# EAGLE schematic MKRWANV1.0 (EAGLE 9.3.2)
Assembly variants: Chip Antenna, Antenna Connector

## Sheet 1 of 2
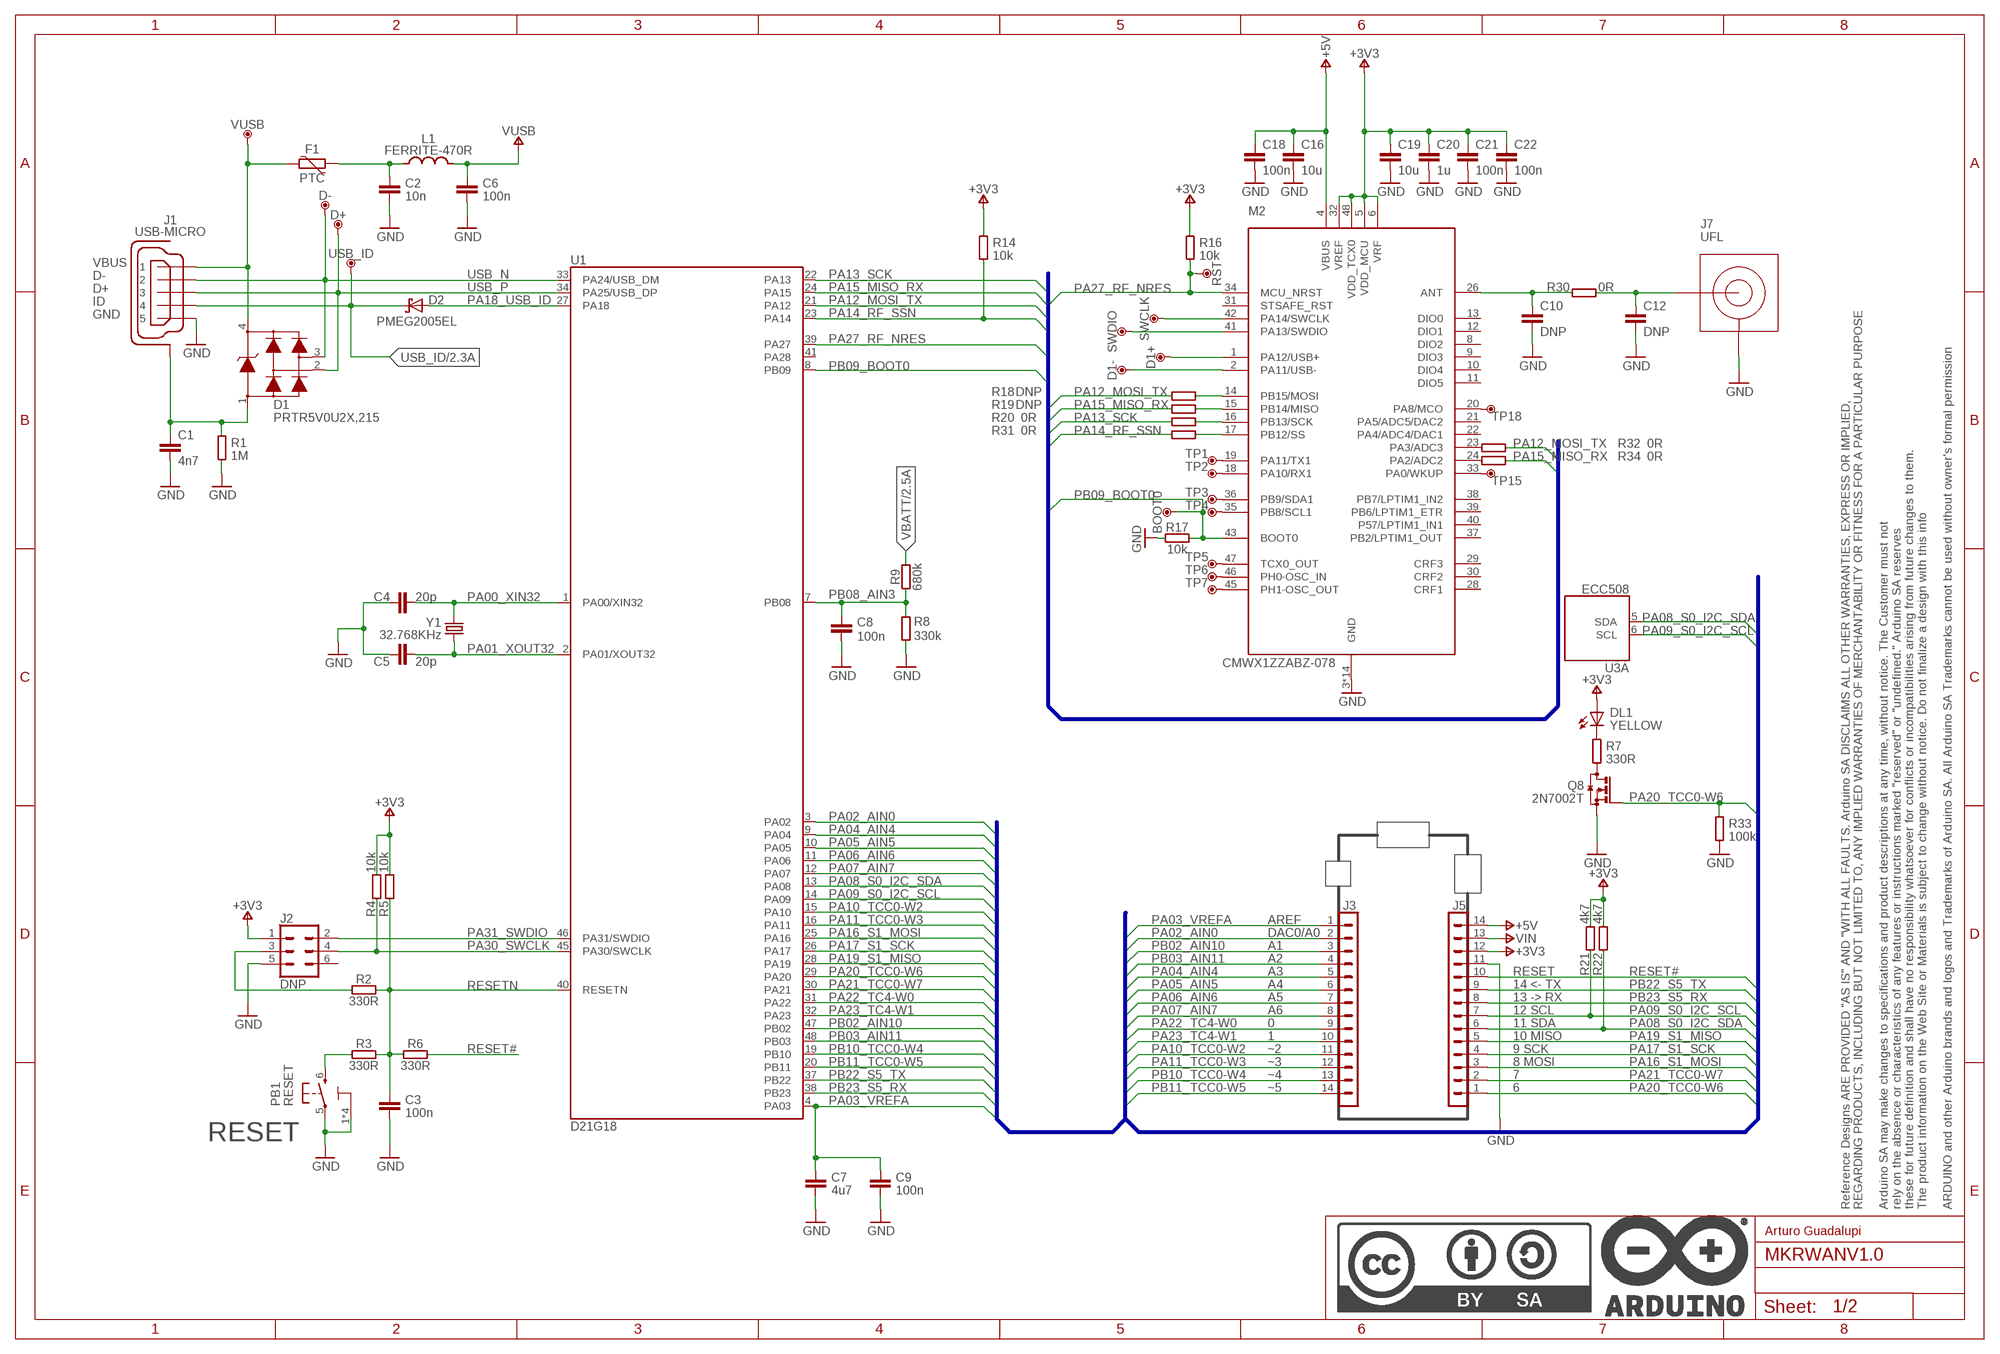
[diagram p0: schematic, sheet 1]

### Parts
BOOT0  DNP  TPTP-1.00MM  [TP-1.00MM]
C1  4n7  C4.7NF-0805  [0805-R2013X50N]
C2  10n  C-10NF-0402  [0402-1005X55N]
C3  100n  C-100NF-0402  [0402-1005X55N]
C4  20p  C-20PF-0402  [0402-1005X55N]
C5  20p  C-20PF-0402  [0402-1005X55N]
C6  100n  C-100NF-0402  [0402-1005X55N]
C7  4u7  C-4.7UF-0402  [0402-1005X55N]
C8  100n  C-100NF-0402  [0402-1005X55N]
C9  100n  C-100NF-0402  [0402-1005X55N]
C10  DNP  CDNP-0402  [0402-1005X55N]
C12  DNP  CDNP-0402  [0402-1005X55N]
C16  10u  C-10UF-0603  [0603-1608X90N]
C18  100n  C-100NF-0402  [0402-1005X55N]
C19  10u  C-10UF-0603  [0603-1608X90N]
C20  1u  C-1UF-0402  [0402-1005X55N]
C21  100n  C-100NF-0402  [0402-1005X55N]
C22  100n  C-100NF-0402  [0402-1005X55N]
D1  PRTR5V0U2X,215  [SOT190P230X110-4N]
D1+  DNP  TPTP-1.00MM  [TP-1.00MM]
D1-  DNP  TPTP-1.00MM  [TP-1.00MM]
D2  PMEG2005EL  [SODFL1008X40N-882D]
D+  DNP  TPTP-1.00MM  [TP-1.00MM]
D-  DNP  TPTP-1.00MM  [TP-1.00MM]
DL1  YELLOW  LED-YELLOW-0603  [LEDC1608X80N-AK]
F1  PTC  [0603-1608X90N]
FRAME1  DNP  A3-FRAME  [FRAME]
J1  USB-MICRO  [ZX62-AB-5PA]
J2  DNP  2X3_SMD_MALE  [2X3_SMT]
J3  DNP  PINHD-1X14-SMTH-SMD  [1X14_SMD_TH]
J5  DNP  PINHD-1X14-SMTH-SMD  [1X14_SMD_TH]
J7  UFL  [U.FL-R-SMT-1(60)]
L1  FERRITE-470R  [0603-1608X90N@1]
M2  CMWX1ZZABZ-078  [CMWX1ZZABZ-078]
PB1  RESET  TACTILE1  [C&K_PTS820_NO_HOLES]
Q8  2N7002T  [SOTFL50P160X78-3]
R1  1M  R-1M-0402  [0402-1005X55N]
R2  330R  R-330R-0402  [0402-1005X55N]
R3  330R  R-330R-0402  [0402-1005X55N]
R4  10k  R-10K-0402  [0402-1005X55N]
R5  10k  R-10K-0402  [0402-1005X55N]
R6  330R  R-330R-0402  [0402-1005X55N]
R7  330R  R-330R-0402  [0402-1005X55N]
R8  330k  R-330K-0402  [0402-1005X55N]
R9  680k  R-680K-0402  [0402-1005X55N]
R14  10k  R-10K-0402  [0402-1005X55N]
R16  10k  R-10K-0402  [0402-1005X55N]
R17  10k  R-10K-0402  [0402-1005X55N]
R18  DNP  R-DNP-0402  [0402-1005X55N]
R19  DNP  R-DNP-0402  [0402-1005X55N]
R20  0R  R-0R-0402  [0402-1005X55N]
R21  4k7  R-4K7-0402  [0402-1005X55N]
R22  4k7  R-4K7-0402  [0402-1005X55N]
R30  0R  R-0R-0402  [0402-1005X55N]
R31  0R  R-0R-0402  [0402-1005X55N]
R32  0R  R-0R-0402  [0402-1005X55N]
R33  100k  R-100K-0402  [0402-1005X55N]
R34  0R  R-0R-0402  [0402-1005X55N]
RST  DNP  TPTP-1.00MM  [TP-1.00MM]
SWCLK  DNP  TPTP-1.00MM  [TP-1.00MM]
SWDIO  DNP  TPTP-1.00MM  [TP-1.00MM]
TP1  DNP  TPTP-0.5MM  [TP-0.50MM]
TP2  DNP  TPTP-0.5MM  [TP-0.50MM]
TP3  DNP  TPTP-0.5MM  [TP-0.50MM]
TP4  DNP  TPTP-0.5MM  [TP-0.50MM]
TP5  DNP  TPTP-0.5MM  [TP-0.50MM]
TP6  DNP  TPTP-0.5MM  [TP-0.50MM]
TP7  DNP  TPTP-0.5MM  [TP-0.50MM]
TP15  DNP  TPTP-0.5MM  [TP-0.50MM]
TP18  DNP  TPTP-0.5MM  [TP-0.50MM]
U1  D21G18  ATSAMD21G18A-48QFN  [QFN50P700X700X90-49XN-EPSQ515]
U3  ECC508  ATECC508A-MAHDA-T8-UDFN  [SON50P300X200X60-9N-EP160X140]
USB_ID  DNP  TPTP-1.00MM  [TP-1.00MM]
VUSB  DNP  TPTP-1.00MM  [TP-1.00MM]
Y1  32.768KHz  32.768KHZ  [ABS07]

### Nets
+3V3: C19.1 C20.1 C21.1 C22.1 DL1.A J2.1 J5.12 M2.5(VDD_MCU) M2.6(VRF) M2.32(VREF) M2.48(VDD_TCX0) R4.2 R5.2 R14.2 R16.2 R21.2 R22.2 ; also sheet 2
+5V: C16.1 C18.1 J5.14 M2.4(VBUS) ; also sheet 2
GND: C1.2 C2.2 C3.2 C4.1 C5.1 C6.2 C7.2 C8.2 C9.2 C10.2 C12.2 C16.2 C18.2 C19.2 C20.2 C21.2 C22.2 J1.5 J2.5 J5.11 J7.GND1(GND) J7.GND2(GND) M2.3(GND) M2.7(GND) M2.25(GND) M2.27(GND) M2.44(GND) M2.49(GND) M2.50(GND) M2.51(GND) M2.52(GND) M2.53(GND) M2.54(GND) M2.55(GND) M2.56(GND) M2.57(GND) PB1.1 PB1.2 PB1.3 PB1.4 PB1.5 Q8.S R1.1 R8.1 R17.1 R33.1 ; also sheet 2
N17650912: D1.4 F1.2 J1.1 VUSB.X
N17658775: PB1.6 R3.1
N$1: C1.1 D1.1 J1.6(SH) J1.7(SH) J1.8(SH) J1.9(SH) J1.10(SH) J1.11(SH) R1.2
N$2: C2.1 F1.1 L1.1
N$3: DL1.C R7.2
N$4: J2.3 R2.1
N$5: M2.24(PA2/ADC2) R34.1
N$6: Q8.D R7.1
N$7: M2.23(PA3/ADC3) R32.1
N$9: M2.19(PA11/TX1) TP1.X
N$10: M2.14(PB15/MOSI) R18.1
N$11: M2.15(PB14/MISO) R19.1
N$13: M2.16(PB13/SCK) R20.1
N$14: M2.17(PB12/SS) R31.1
N$15: M2.41(PA13/SWDIO) SWDIO.X
N$16: M2.42(PA14/SWCLK) SWCLK.X
N$17: C12.1 J7.SIG R30.2
N$18: D1+.X M2.1(PA12/USB+)
N$19: D1-.X M2.2(PA11/USB-)
N$20: M2.18(PA10/RX1) TP2.X
N$21: M2.36(PB9/SDA1) TP3.X
N$22: M2.35(PB8/SCL1) TP4.X
N$23: M2.47(TCX0_OUT) TP5.X
N$24: M2.46(PH0-OSC_IN) TP6.X
N$25: M2.45(PH1-OSC_OUT) TP7.X
N$33: M2.33(PA0/WKUP) TP15.X
N$36: M2.20(PA8/MCO) TP18.X
N$38: C10.1 M2.26(ANT) R30.1
PA00_XIN32: C4.2 U1.1(PA00/XIN32) Y1.2
PA01_XOUT32: C5.2 U1.2(PA01/XOUT32) Y1.1
PA02_AIN0: J3.2 U1.3(PA02)
PA03_VREFA: C7.1 C9.1 J3.1 U1.4(PA03)
PA04_AIN4: J3.5 U1.9(PA04)
PA05_AIN5: J3.6 U1.10(PA05)
PA06_AIN6: J3.7 U1.11(PA06)
PA07_AIN7: J3.8 U1.12(PA07)
PA08_S0_I2C_SDA: J5.6 R22.1 U1.13(PA08) U3.5(A:SDA)
PA09_S0_I2C_SCL: J5.7 R21.1 U1.14(PA09) U3.6(A:SCL)
PA10_TCC0-W2: J3.11 U1.15(PA10)
PA11_TCC0-W3: J3.12 U1.16(PA11)
PA12_MOSI_TX: R18.2 R32.2 U1.21(PA12)
PA13_SCK: R20.2 U1.22(PA13)
PA14_RF_SSN: R14.1 R31.2 U1.23(PA14)
PA15_MISO_RX: R19.2 R34.2 U1.24(PA15)
PA16_S1_MOSI: J5.3 U1.25(PA16)
PA17_S1_SCK: J5.4 U1.26(PA17)
PA18_USB_ID: D2.A U1.27(PA18)
PA19_S1_MISO: J5.5 U1.28(PA19)
PA20_TCC0-W6: J5.1 Q8.G R33.2 U1.29(PA20)
PA21_TCC0-W7: J5.2 U1.30(PA21)
PA22_TC4-W0: J3.9 U1.31(PA22)
PA23_TC4-W1: J3.10 U1.32(PA23)
PA27_RF_NRES: M2.34(MCU_NRST) R16.1 RST.X U1.39(PA27)
PA30_SWCLK: J2.4 R4.1 U1.45(PA30/SWCLK)
PA31_SWDIO: J2.2 U1.46(PA31/SWDIO)
PB02_AIN10: J3.3 U1.47(PB02)
PB03_AIN11: J3.4 U1.48(PB03)
PB08_AIN3: C8.1 R8.2 R9.1 U1.7(PB08)
PB09_BOOT0: BOOT0.X M2.43(BOOT0) R17.2 U1.8(PB09)
PB10_TCC0-W4: J3.13 U1.19(PB10)
PB11_TCC0-W5: J3.14 U1.20(PB11)
PB22_S5_TX: J5.9 U1.37(PB22)
PB23_S5_RX: J5.8 U1.38(PB23)
RESET#: J5.10 R6.2
RESETN: C3.1 R2.2 R3.2 R5.1 R6.1 U1.40(RESETN)
USB_ID: D2.C J1.4 USB_ID.X ; also sheet 2
USB_N: D1.3 D-.X J1.2 U1.33(PA24/USB_DM)
USB_P: D1.2 D+.X J1.3 U1.34(PA25/USB_DP)
VBATT: R9.2 ; also sheet 2
VIN: J5.13 ; also sheet 2
VUSB: C6.1 L1.2 ; also sheet 2
Unconnected: J2.6 M2.8(DIO2) M2.9(DIO3) M2.10(DIO4) M2.11(DIO5) M2.12(DIO1) M2.13(DIO0) M2.21(PA5/ADC5/DAC2) M2.22(PA4/ADC4/DAC1) M2.28(CRF1) M2.29(CRF3) M2.30(CRF2) M2.31(STSAFE_RST) M2.37(PB2/LPTIM1_OUT) M2.38(PB7/LPTIM1_IN2) M2.39(PB6/LPTIM1_ETR) M2.40(P57/LPTIM1_IN1) U1.41(PA28)

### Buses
PA03_VREFA,PA02_AIN0,PB02_AIN10,PB03_AIN11,PA04_AIN4,PA05_AIN5,PA06_AIN6,PA07_AIN7,PA22_TC4-W0,PA23_TC4-W1,PA10_TCC0-W2,PA11_TCC0-W3,PB10_TCC0-W4,PB11_TCC0-W5,PA20_TCC0-W6,PA21_TCC0-W7,PA16_S1_MOSI,PA17_S1_SCK,PA19_S1_MISO,PA08_S0_I2C_SDA,PA09_S0_I2C_SCL,PB23_S5_RX,PB22_S5_TX,RESET#
B$1

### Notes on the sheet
- AREF
- DAC0/A0
- A1
- A2
- A3 | RESET
- A4 | 14 <- TX
- A5 | 13 -> RX
- A6 | 12 SCL
- 0 | 11 SDA
- 1 | 10 MISO
- ~2 | 9 SCK
- ~3 | 8 MOSI
- ~4 | 7
- ~5 | 6
- RESET
- Arturo Guadalupi

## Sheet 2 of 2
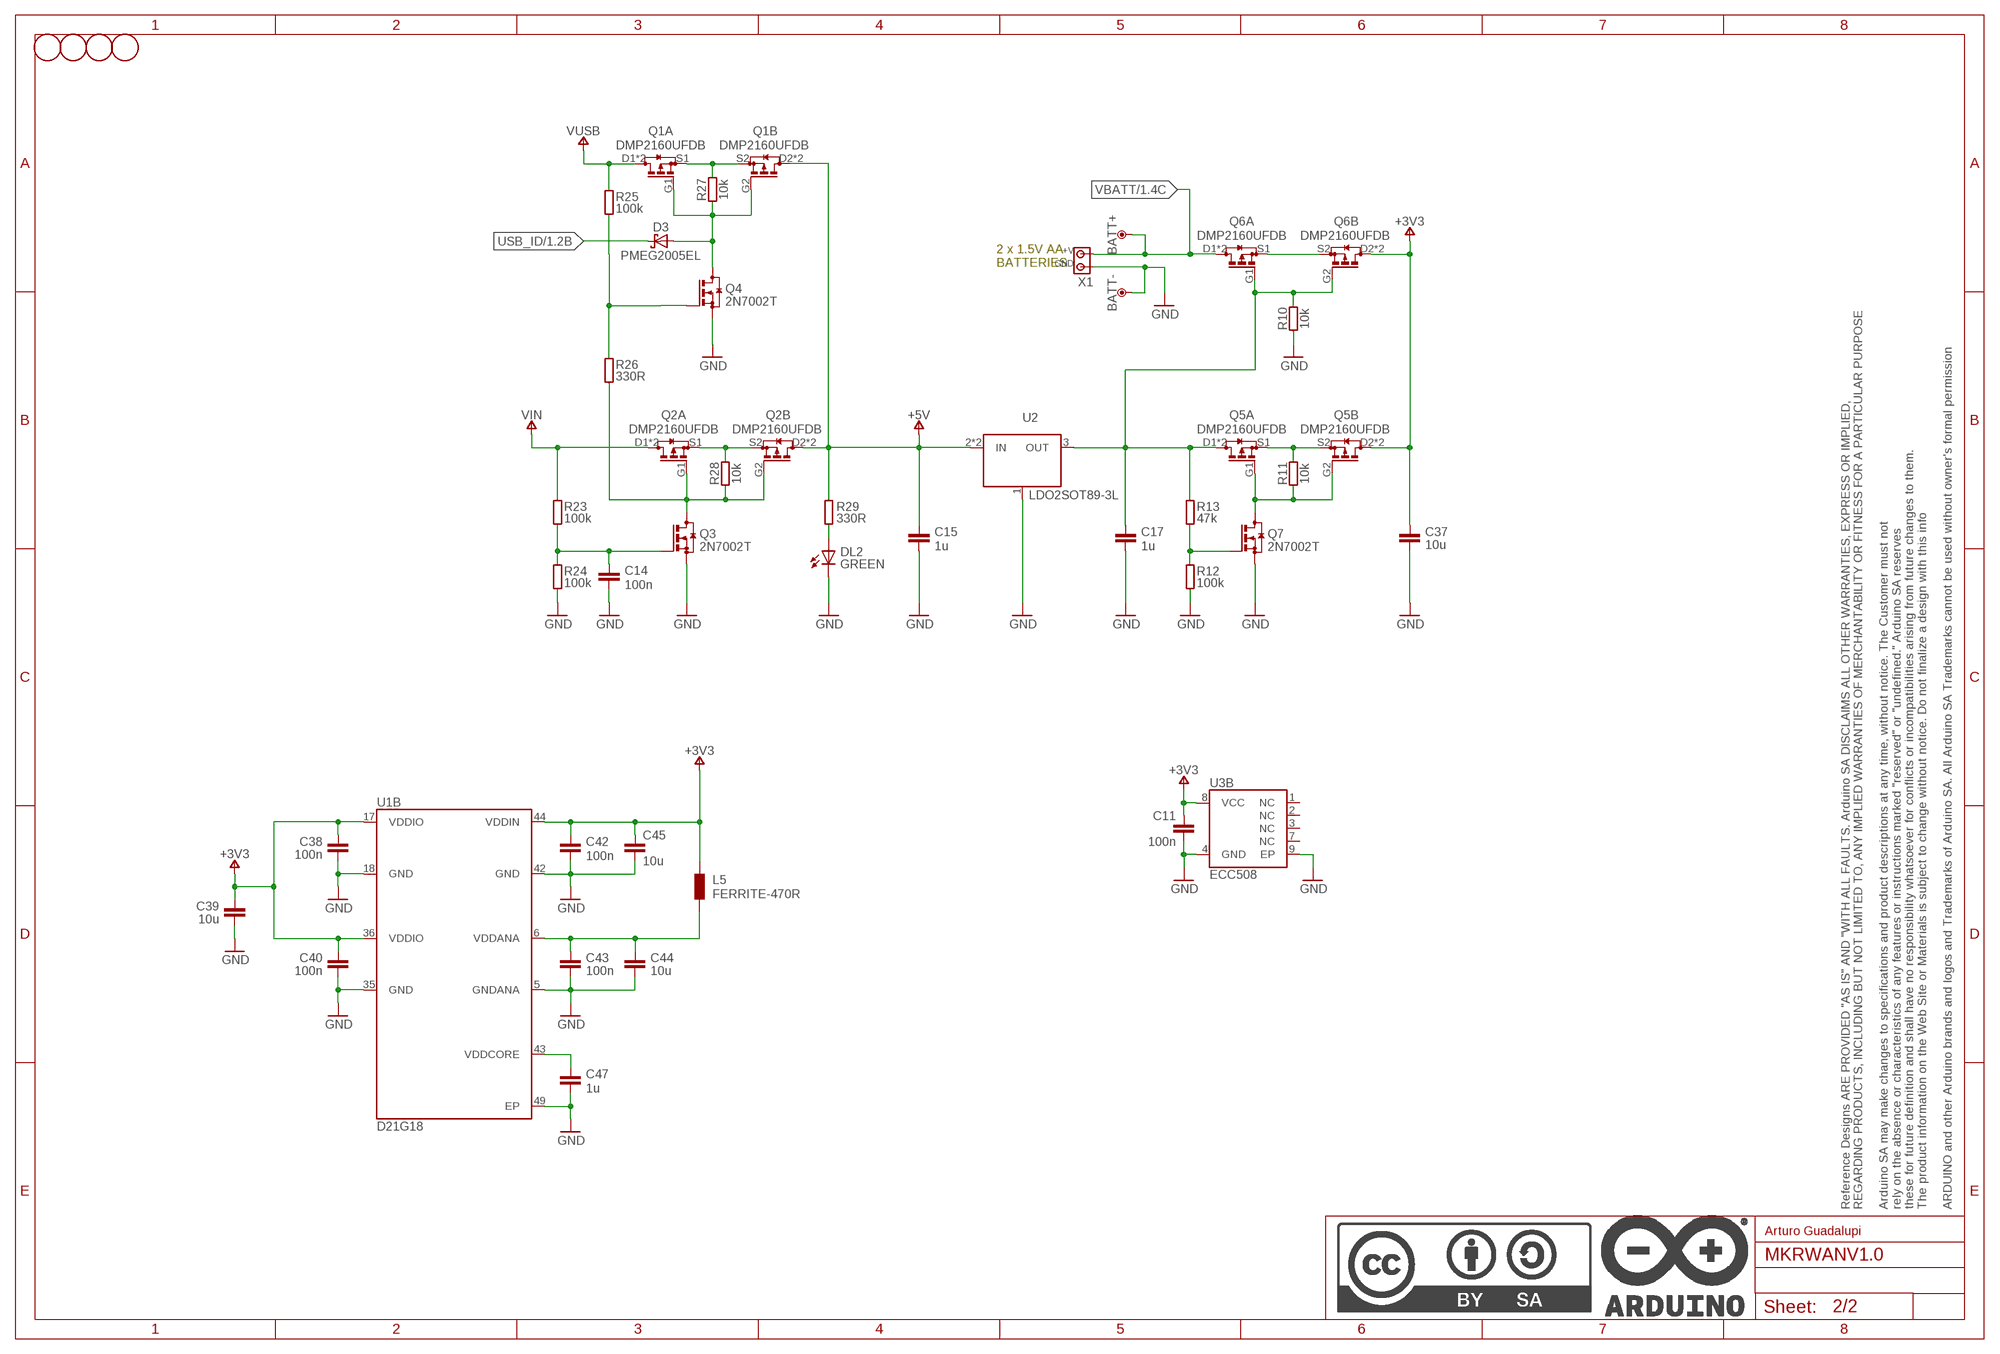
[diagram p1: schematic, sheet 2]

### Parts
BATT+  DNP  TPTP-1.00MM  [TP-1.00MM]
BATT-  DNP  TPTP-1.00MM  [TP-1.00MM]
C11  100n  C-100NF-0402  [0402-1005X55N]
C14  100n  C-100NF-0402  [0402-1005X55N]
C15  1u  C-1UF-0402  [0402-1005X55N]
C17  1u  C-1UF-0402  [0402-1005X55N]
C37  10u  C-10UF-0603  [0603-1608X90N]
C38  100n  C-100NF-0402  [0402-1005X55N]
C39  10u  C-10UF-0603  [0603-1608X90N]
C40  100n  C-100NF-0402  [0402-1005X55N]
C42  100n  C-100NF-0402  [0402-1005X55N]
C43  100n  C-100NF-0402  [0402-1005X55N]
C44  10u  C-10UF-0603  [0603-1608X90N]
C45  10u  C-10UF-0603  [0603-1608X90N]
C47  1u  C-1UF-0402  [0402-1005X55N]
D3  PMEG2005EL  [SODFL1008X40N-882D]
DL2  GREEN  LED-GREEN-0603  [LEDC1608X80N-AK]
FD1  DNP  FIDUCIAL-1.5MM  [FD-1-1.5]
FD2  DNP  FIDUCIAL-1.5MM  [FD-1-1.5]
FD3  DNP  FIDUCIAL-1.5MM  [FD-1-1.5]
FD4  DNP  FIDUCIAL-1.5MM  [FD-1-1.5]
FRAME2  DNP  A3-FRAME  [FRAME]
L5  FERRITE-470R  [0603-1608X90N@1]
Q1  DMP2160UFDB  [PWR_SC70]
Q2  DMP2160UFDB  [PWR_SC70]
Q3  2N7002T  [SOTFL50P160X78-3]
Q4  2N7002T  [SOTFL50P160X78-3]
Q5  DMP2160UFDB  [PWR_SC70]
Q6  DMP2160UFDB  [PWR_SC70]
Q7  2N7002T  [SOTFL50P160X78-3]
R10  10k  R-10K-0402  [0402-1005X55N]
R11  10k  R-10K-0402  [0402-1005X55N]
R12  100k  R-100K-0402  [0402-1005X55N]
R13  47k  R-47K-0402  [0402-1005X55N]
R23  100k  R-100K-0402  [0402-1005X55N]
R24  100k  R-100K-0402  [0402-1005X55N]
R25  100k  R-100K-0402  [0402-1005X55N]
R26  330R  R-330R-0402  [0402-1005X55N]
R27  10k  R-10K-0402  [0402-1005X55N]
R28  10k  R-10K-0402  [0402-1005X55N]
R29  330R  R-330R-0402  [0402-1005X55N]
U2  LDO2SOT89-3L  [SOT89-3L]
X1  SCREW2X2.54  [SCREW2]

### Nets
+3V3: C11.1 C37.1 C38.1 C39.1 C40.1 C42.1 C45.1 L5.1 Q5.D2'(B:D) Q5.D2(B:D) Q6.D2'(B:D) Q6.D2(B:D) U1.17(VDDIO) U1.36(VDDIO) U1.44(VDDIN) U3.8(B:VCC) ; also sheet 1
+5V: C15.1 Q1.D2'(B:D) Q1.D2(B:D) Q2.D2'(B:D) Q2.D2(B:D) R29.2 U2.2(IN) U2.TH(IN) ; also sheet 1
GND: BATT-.X C11.2 C14.2 C15.2 C17.2 C37.2 C38.2 C39.2 C40.2 C42.2 C43.2 C44.2 C45.2 C47.2 DL2.C Q3.S Q4.S Q7.S R10.1 R12.1 R24.1 U1.5(GNDANA) U1.18(GND) U1.35(GND) U1.42(GND) U1.49(EP) U2.1(GND/ADJ) U3.4(B:GND) U3.9(B:EP) X1.GND ; also sheet 1
N1: Q5.S1(A:S) Q5.S2(B:S) R11.2
N2: Q5.G1(A:G) Q5.G2(B:G) Q7.D R11.1
N3: Q7.G R12.2 R13.1
N17690335: Q1.S1(A:S) Q1.S2(B:S) R27.2
N17690346: D3.A Q1.G1(A:G) Q1.G2(B:G) Q4.D R27.1
N17690381: Q4.G R25.1 R26.2
N17690821: Q2.S1(A:S) Q2.S2(B:S) R28.2
N17690840: Q2.G1(A:G) Q2.G2(B:G) Q3.D R26.1 R28.1
N17690878: C14.1 Q3.G R23.1 R24.2
N17834267: DL2.A R29.1
N17852357: C43.1 C44.1 L5.2 U1.6(VDDANA)
N$8: C17.1 Q5.D1'(A:D) Q5.D1(A:D) Q6.G1(A:G) Q6.G2(B:G) R10.2 R13.2 U2.3(OUT)
N$12: Q6.S1(A:S) Q6.S2(B:S)
N$46: C47.1 U1.43(VDDCORE)
USB_ID: D3.C ; also sheet 1
VBATT: BATT+.X Q6.D1'(A:D) Q6.D1(A:D) X1.V+ ; also sheet 1
VIN: Q2.D1'(A:D) Q2.D1(A:D) R23.2 ; also sheet 1
VUSB: Q1.D1'(A:D) Q1.D1(A:D) R25.2 ; also sheet 1
Unconnected: U3.1(B:NC) U3.2(B:NC) U3.3(B:NC) U3.7(B:NC)

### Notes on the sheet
- 2 x 1.5V AA
  BATTERIES
- Arturo Guadalupi

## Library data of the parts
BATT+ BATT- BOOT0 D1+ D1- D+ D- RST SWCLK SWDIO TP1-TP7 TP15 TP18 USB_ID VUSB = Arduino-utility:TP: Testpoint; DATASHEET: DNP; DISTRIBUTOR-LINK: DNP; DISTRIBUTOR-PN: DNP; MANUFACTURER: DNP; MANUFACTURER-PN: DNP
C1 = Arduino-rcl:C: SMD Capacitor; DATASHEET: http://www.kemet.com/Lists/ProductCatalog/Attachments/40/KEM_C1010_X7R_HV_SMD.pdf; DISTRIBUTOR-LINK: www.kemet.com/docfinder?Partnumber=C0805C472KDRACTU; DISTRIBUTOR-PN: 399-6738-1-ND; MANUFACTURER: Kemet; MANUFACTURER-PN: C0805C472KDRACTU
C2 = Arduino-rcl:C: SMD Capacitor; DATASHEET: http://search.murata.co.jp/Ceramy/image/img/A01X/partnumbering_e_01.pdf; DISTRIBUTOR-LINK: http://www.digikey.com/product-detail/en/murata-electronics-north-america/GRM155R71H103KA88J/490-6351-1-ND/3845548; DISTRIBUTOR-PN: 490-6351-1-ND; MANUFACTURER: Murata; MANUFACTURER-PN: GRM155R71H103KA88J
C3 C6 C8 C9 C11 C14 C18 C21 C22 C38 C40 C42 C43 = Arduino-rcl:C: SMD Capacitor; DATASHEET: http://www.tdk.com/pdf/TDKMLCCCapRange.pdf; DISTRIBUTOR-LINK: http://www.digikey.com/product-detail/en/tdk-corporation/C1005X5R1H104K050BB/445-5942-1-ND/2443982; DISTRIBUTOR-PN: 445-5942-1-ND; MANUFACTURER: TDK; MANUFACTURER-PN: C1005X5R1H104K050BB
C4 C5 = Arduino-rcl:C: SMD Capacitor; DATASHEET: http://www.kemet.com/docfinder?Partnumber=CBR04C200J5GAC; DISTRIBUTOR-LINK: http://www.digikey.com/product-detail/en/kemet/CBR04C200J5GAC/399-6173-1-ND/2732143; DISTRIBUTOR-PN: 399-6173-1-ND; MANUFACTURER: Kemet; MANUFACTURER-PN: CBR04C200J5GAC
C7 = Arduino-rcl:C: SMD Capacitor; DATASHEET: http://search.murata.co.jp/Ceramy/image/img/A01X/partnumbering_e_01.pdf; DISTRIBUTOR-LINK: http://www.digikey.com/product-detail/en/murata-electronics-north-america/GRM155R60J475ME47D/490-5915-1-ND/3719860; DISTRIBUTOR-PN: 490-5915-1-ND; MANUFACTURER: Murata; MANUFACTURER-PN: GRM155R60J475ME47D
C10 C12 = Arduino-rcl:C: SMD Capacitor; DATASHEET: DNP; DISTRIBUTOR-LINK: DNP; DISTRIBUTOR-PN: DNP; MANUFACTURER: DNP; MANUFACTURER-PN: DNP
C15 C17 C20 C47 = Arduino-rcl:C: SMD Capacitor; DATASHEET: http://search.murata.co.jp/Ceramy/image/img/A01X/partnumbering_e_01.pdf; DISTRIBUTOR-LINK: http://www.digikey.com/product-detail/en/murata-electronics-north-america/GRM155R61E105KA12D/490-10017-1-ND/5026367; DISTRIBUTOR-PN: 490-10017-1-ND; MANUFACTURER: Murata; MANUFACTURER-PN: GRM155R61E105KA12D
C16 C19 C37 C39 C44 C45 = Arduino-rcl:C: SMD Capacitor; DATASHEET: http://www.murata.com/~/media/webrenewal/support/library/catalog/products/capacitor/mlcc/c02e.pdf; DISTRIBUTOR-LINK: http://www.digikey.com/product-search/en?keywords=490-10728-1-ND; DISTRIBUTOR-PN: 490-10728-1-ND; MANUFACTURER: Murata; MANUFACTURER-PN: GRM188R61C106KAALD
D1 = Arduino-diodes:PRTR5V0U2X,215: USB ESD protection; DATASHEET: http://www.nxp.com/documents/data_sheet/PRTR5V0U2X.pdf; DISTRIBUTOR-LINK: http://www.digikey.com/product-detail/en/nxp-semiconductors/PRTR5V0U2X,215/568-4140-1-ND/1589981; DISTRIBUTOR-PN: 568-4140-1-ND; MANUFACTURER: NXP; MANUFACTURER-PN: PRTR5V0U2X,215
D2 D3 = Arduino-diodes:PMEG2005EL: DIODE SCHOTTKY 20V 500MA SOD882; DATASHEET: http://www.nxp.com/documents/data_sheet/PMEG2005EL.pdf; DISTRIBUTOR-LINK: http://www.digikey.com/product-detail/en/nxp-semiconductors/PMEG2005EL,315/568-6754-1-ND/2676794; DISTRIBUTOR-PN: 568-6754-1-ND; MANUFACTURER: NXP; MANUFACTURER-PN: PMEG2005EL,315
DL1 = Arduino-diodes:LED: LED; DATASHEET: http://media.digikey.com/pdf/Data%20Sheets/Avago%20PDFs/HSMz-Czzz.pdf; DISTRIBUTOR-LINK: http://www.digikey.com/product-detail/en/broadcom-limited/HSMY-C190/516-1424-1-ND/637748; DISTRIBUTOR-PN: 516-1424-1-ND; MANUFACTURER: Avago; MANUFACTURER-PN: HSMY-C190
DL2 = Arduino-diodes:LED: LED; DATASHEET: http://media.digikey.com/pdf/Data%20Sheets/Avago%20PDFs/HSMz-Czzz.pdf; DISTRIBUTOR-LINK: http://www.digikey.com/product-detail/en/broadcom-limited/HSMG-C190/516-1425-1-ND/637749; DISTRIBUTOR-PN: 516-1425-1-ND; MANUFACTURER: Avago; MANUFACTURER-PN: HSMG-C190
F1 = Arduino-rcl:PTC: SMD PTC; DATASHEET: http://www.bourns.com/docs/Product-Datasheets/mffsmf.pdf; DISTRIBUTOR-LINK: http://www.digikey.com/product-detail/en/bourns-inc/MF-FSMF050X-2/MF-FSMF050X-2CT-ND/2039389; DISTRIBUTOR-PN: MF-FSMF050X-2CT-ND; MANUFACTURER: Bourns Inc; MANUFACTURER-PN: MF-FSMF050X-2
FD1-FD4 = Arduino-utility:FIDUCIAL: Fiducial mount; DATASHEET: DNP; DISTRIBUTOR-LINK: DNP; DISTRIBUTOR-PN: DNP; MANUFACTURER: DNP; MANUFACTURER-PN: DNP
FRAME1 FRAME2 = Arduino-utility:A3-FRAME; CODE-ARDUINO: DNP; DATASHEET: DNP; DISTRIBUTOR-LINK: DNP; DISTRIBUTOR-PN: DNP; MANUFACTURER: DNP; MANUFACTURER-PN: DNP; NOTE: DNP
J1 = Arduino-connectors:USB-MICRO: USB - micro AB USB 2.0 Receptacle Connector 5 Position Surface Mount, Right Angle, Horizontal; DATASHEET: https://www.hirose.com/product/en/download_file/key_name/ZX/category/Catalog/doc_file_id/31704/?file_category_id=4&item_id=13&is_series=1; DISTRIBUTOR-LINK: http://www.digikey.com/product-detail/en/hirose-electric-co-ltd/ZX62-AB-5PA(31)/H125279CT-ND/5994741; DISTRIBUTOR-PN: H125279CT-ND; MANUFACTURER: Hirose; MANUFACTURER-PN: ZX62-AB-5PA(31)
J2 = Arduino-connectors:2X3_SMD_MALE: SMD connector; DATASHEET: DNP; DISTRIBUTOR-LINK: DNP; DISTRIBUTOR-PN: DNP; MANUFACTURER: DNP; MANUFACTURER-PN: DNP
J3 J5 = Arduino-connectors:PINHD-1X14-SM: PIN HEADER; DATASHEET: -; DISTRIBUTOR-LINK: -; DISTRIBUTOR-PN: -; MANUFACTURER: ELDECO; MANUFACTURER-PN: FH254114DF08500T
J7 = Arduino-connectors:UFL: U.FL, Ultra Miniature Coaxial Connector Receptacle, Male Pin 50 Ohm Surface Mount Solder; DATASHEET: http://media.digikey.com/pdf/Data%20Sheets/Hirose%20PDFs/UFL%20Series.pdf; DISTRIBUTOR-LINK: http://www.digikey.com/product-search/en?keywords=U.FL-R-SMT-1(60); DISTRIBUTOR-PN: U.FL-R-SMT-1(60)-ND; MANUFACTURER: Hirose; MANUFACTURER-PN: U.FL-R-SMT-1(60)
L1 = Arduino-rcl:FERRITE-470R: FERRITE BEAD 470 OHM 0603 1LN; DATASHEET: http://search.murata.co.jp/Ceramy/image/img/PDF/ENG/L0110S0100BLM18P.pdf; DISTRIBUTOR-LINK: http://www.digikey.com/product-detail/en/murata-electronics-north-america/BLM18PG471SN1D/490-5223-1-ND/1948399; DISTRIBUTOR-PN: 490-5223-1-ND; MANUFACTURER: Murata; MANUFACTURER-PN: BLM18PG471SN1D
L5 = Arduino-rcl:FERRITE: FERRITE BEAD 470 OHM 0603 1LN; DATASHEET: http://search.murata.co.jp/Ceramy/image/img/PDF/ENG/L0110S0100BLM18P.pdf; DISTRIBUTOR-LINK: http://www.digikey.com/product-detail/en/murata-electronics-north-america/BLM18PG471SN1D/490-5223-1-ND/1948399; DISTRIBUTOR-PN: 490-5223-1-ND; MANUFACTURER: Murata; MANUFACTURER-PN: BLM18PG471SN1D
M2 = Arduino-ucs&SoCs:CMWX1ZZABZ-078; DATASHEET: https://www.arrow.altech.co.za/sites/arrow/files/Murata%20LoRa%20Module%20Preliminary%20Datasheet%20SP-ABZ-G.PDF; DISTRIBUTOR-LINK: https://www.digikey.com/product-detail/en/murata-electronics-north-america/CMWX1ZZABZ-078/490-16143-1-ND/6834151; DISTRIBUTOR-PN: 490-16143-1-ND; MANUFACTURER: Murata; MANUFACTURER-PN: CMWX1ZZABZ-078
PB1 = Arduino-pushbuttons:TACTILE1: Tactile Switch SPST-NO Top Actuated Surface Mount; DATASHEET: http://www.ckswitches.com/media/1474/pts820.pdf; DISTRIBUTOR-LINK: http://www.digikey.com/product-detail/en/c-k-components/PTS820%20J25K%20SMTR%20LFS/PTS820%20J25K%20SMTR%20LFS-ND/4142165; DISTRIBUTOR-PN: PTS820 J25K SMTR LFS-ND; MANUFACTURER: C&K; MANUFACTURER-PN: PTS820 J25K SMTR LFS
Q1 Q2 Q5 Q6 = Arduino-transistors:DMP2160UFDB: MOSFET 2P-CH 20V 3.8A 6UDFN; DATASHEET: http://www.diodes.com/_files/datasheets/ds31643.pdf; DISTRIBUTOR-LINK: http://www.digikey.com/product-detail/en/diodes-incorporated/DMP2160UFDB-7/DMP2160UFDB-7DI-ND/4249940; DISTRIBUTOR-PN: DMP2160UFDB-7DI-ND; MANUFACTURER: Diodes Inc; MANUFACTURER-PN: DMP2160UFDB-7
Q3 Q4 Q7 Q8 = Arduino-transistors:2N7002T: MOSFET N-CH 60V 115MA SOT-523; DATASHEET: http://www.diodes.com/_files/datasheets/ds30301.pdf; DISTRIBUTOR-LINK: http://www.digikey.com/product-detail/en/diodes-incorporated/2N7002T-7-F/2N7002T-FDICT-ND/815290; DISTRIBUTOR-PN: 2N7002T-FDICT-ND; MANUFACTURER: Diodes Incorporated; MANUFACTURER-PN: 2N7002T-7-F
R1 = Arduino-rcl:R: SMD Resistor; DATASHEET: www.yageo.com.tw/exep/pages/download/literatures/PYu-R_INT-thick_7.pdf; DISTRIBUTOR-LINK: http://www.digikey.com/product-detail/en/yageo/RC0402JR-07330RL/311-330JRCT-ND/729412; DISTRIBUTOR-PN: 311-330JRCT-ND; MANUFACTURER: Yageo; MANUFACTURER-PN: RC0402JR-07330RL
R2 R3 R6 R7 R26 R29 = Arduino-rcl:R: SMD Resistor; DATASHEET: www.yageo.com.tw/exep/pages/download/literatures/PYu-R_INT-thick_7.pdf; DISTRIBUTOR-LINK: http://www.digikey.com/product-detail/en/yageo/RC0402FR-07330RL/311-330LRCT-ND/729541; DISTRIBUTOR-PN: 311-330LRCT-ND; MANUFACTURER: Yageo; MANUFACTURER-PN: RC0402FR-07330RL
R4 R5 R10 R11 R14 R16 R17 R27 R28 = Arduino-rcl:R: SMD Resistor; DATASHEET: www.yageo.com.tw/exep/pages/download/literatures/PYu-R_INT-thick_7.pdf; DISTRIBUTOR-LINK: http://www.digikey.com/product-detail/en/yageo/RC0402FR-0710KL/311-10.0KLRCT-ND/729470; DISTRIBUTOR-PN: 311-10.0KLRCT-ND; MANUFACTURER: Yageo; MANUFACTURER-PN: RC0402FR-0710KL
R8 = Arduino-rcl:R: SMD Resistor; DATASHEET: www.yageo.com.tw/exep/pages/download/literatures/PYu-R_INT-thick_7.pdf; DISTRIBUTOR-LINK: http://www.digikey.com/product-detail/en/yageo/RC0402JR-07330KL/311-330KJRCT-ND/729413; DISTRIBUTOR-PN: 311-330KJRCT-ND; MANUFACTURER: Yageo; MANUFACTURER-PN: RC0402JR-07330KL
R9 = Arduino-rcl:R: SMD Resistor; DATASHEET: www.yageo.com.tw/exep/pages/download/literatures/PYu-R_INT-thick_7.pdf; DISTRIBUTOR-LINK: http://www.digikey.it/product-detail/it/yageo/RC0402JR-07680KL/311-680KJRTR-ND/726501; DISTRIBUTOR-PN: 311-680KJRTR-ND; MANUFACTURER: Yageo; MANUFACTURER-PN: RC0402JR-07680KL
R12 R23-R25 R33 = Arduino-rcl:R: SMD Resistor; DATASHEET: www.yageo.com.tw/exep/pages/download/literatures/PYu-R_INT-thick_7.pdf; DISTRIBUTOR-LINK: http://www.digikey.com/product-detail/en/yageo/RC0402FR-07100KL/311-100KLRCT-ND/729473; DISTRIBUTOR-PN: 311-100KLRCT-ND; MANUFACTURER: Yageo; MANUFACTURER-PN: RC0402FR-07100KL
R13 = Arduino-rcl:R: SMD Resistor; DATASHEET: www.yageo.com.tw/exep/pages/download/literatures/PYu-R_INT-thick_7.pdf; DISTRIBUTOR-LINK: http://www.digikey.com/product-detail/en/yageo/RC0402JR-0747KL/311-47KJRCT-ND/729432; DISTRIBUTOR-PN: 311-47KJRCT-ND; MANUFACTURER: Yageo; MANUFACTURER-PN: RC0402JR-0747KL
R18 R19 = Arduino-rcl:R: SMD Resistor; DATASHEET: DNP; DISTRIBUTOR-LINK: DNP; DISTRIBUTOR-PN: DNP; MANUFACTURER: DNP; MANUFACTURER-PN: DNP
R20 R30-R32 R34 = Arduino-rcl:R: SMD Resistor; DATASHEET: www.yageo.com.tw/exep/pages/download/literatures/PYu-R_INT-thick_7.pdf; DISTRIBUTOR-LINK: http://www.digikey.com/product-detail/en/yageo/RC0402FR-070RL/311-0.0LRCT-ND/2827888; DISTRIBUTOR-PN: 311-0.0LRCT-ND; MANUFACTURER: Yageo; MANUFACTURER-PN: RC0402FR-070RL
R21 R22 = Arduino-rcl:R: SMD Resistor; DATASHEET: www.yageo.com.tw/exep/pages/download/literatures/PYu-R_INT-thick_7.pdf; DISTRIBUTOR-LINK: http://www.digikey.com/product-detail/en/yageo/RC0402FR-074K7L/311-4.7KLRCT-ND/2827881; DISTRIBUTOR-PN: 311-4.7KLRCT-ND; MANUFACTURER: Yageo; MANUFACTURER-PN: RC0402FR-074K7L
U1 = Arduino-ucs&SoCs:ATSAMD21G18A-48: ARM® Cortex®-M0+ SAM D21G Microcontroller IC 32-Bit 48MHz 256KB (256K x 8) FLASH 48-TQFP (7x7); DATASHEET: http://www.atmel.com/Images/Atmel-42181-SAM-D21_Datasheet.pdf; DISTRIBUTOR-LINK: http://www.digikey.com/product-detail/en/atmel/ATSAMD21G18A-AUT/ATSAMD21G18A-AUTCT-ND/4878879; DISTRIBUTOR-PN: ATSAMD21G18A-AUTCT-ND; MANUFACTURER: Atmel; MANUFACTURER-PN: ATSAMD21G18A-MU
U2 = Arduino-ICs:LDO2; DATASHEET: http://www.diodes.com/_files/datasheets/AP7215.pdf; DISTRIBUTOR-LINK: http://www.digikey.com/product-detail/en/diodes-incorporated/AP7215-33YG-13/AP7215-33YG-13DICT-ND/2179740; DISTRIBUTOR-PN: AP7215-33YG-13DICT-ND; MANUFACTURER: Diodes Inc; MANUFACTURER-PN: AP7215-33YG-13
U3 = Arduino-ICs:ATECC508A-MAHDA-T: Secure authentication and product validation device, EEPROM, I2C, 2.0 - 5.5V; DATASHEET: http://www.atmel.com/Images/Atmel-8923S-CryptoAuth-ATECC508A-Datasheet-Summary.pdf; DISTRIBUTOR-LINK: http://www.digikey.com/product-detail/en/atmel/ATECC508A-MAHDA-T/ATECC508A-MAHDA-TCT-ND/5213071; DISTRIBUTOR-PN: ATECC508A-MAHDA-TCT-ND; MANUFACTURER: Atmel; MANUFACTURER-PN: ATECC508A-MAHDA-T
X1 = Arduino-connectors:SCREW2X2.54: 2.45 Screw terminal Block; DATASHEET: http://www.on-shore.com/wp-content/uploads/2015/09/ostvnxxa150.pdf; DISTRIBUTOR-LINK: http://www.digikey.com/product-detail/en/on-shore-technology-inc/OSTVN02A150/ED10561-ND/1588862; DISTRIBUTOR-PN: ED10561-ND; MANUFACTURER: On Shore Technology Inc.; MANUFACTURER-PN: OSTVN02A150
Y1 = Arduino-crystals:32.768KHZ: LF crystal; DATASHEET: http://www.abracon.com/Resonators/ABS07.pdf; DISTRIBUTOR-LINK: http://www.digikey.com/product-detail/en/abracon-llc/ABS07-32.768KHZ-T/535-9542-1-ND/1237009; DISTRIBUTOR-PN: 535-9542-1-ND; MANUFACTURER: Abracon LLC; MANUFACTURER-PN: ABS07-32.768KHZ-T

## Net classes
0 default: width 0.25 mm, drill 0.195 mm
